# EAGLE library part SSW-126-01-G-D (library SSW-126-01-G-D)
52 Position, .100" Tiger Buy&trade; Socket Strip Source: Datasheet
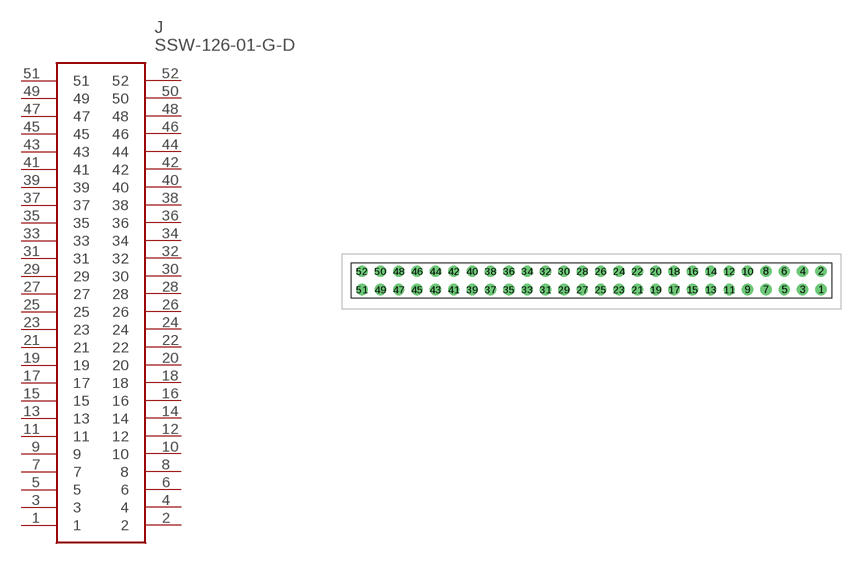
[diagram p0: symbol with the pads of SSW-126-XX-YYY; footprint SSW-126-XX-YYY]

Designator prefix J

## SSW-126-01-G-D (Description: 52 Position, .100&quot; Tiger Buy&trade; Socket Strip; Height: mm; Manufacturer_Name: SAMTEC; Manufacturer_Part_Number: SSW-126-01-G-D; Mouser_Part_Number: 200-SSW12601GD; Mouser_Price-Stock: https://www.mouser.co.uk/ProductDetail/Samtec/SSW-126-01-G-D?qs=rU5fayqh%252BE0Emlk%2F61GTGg%3D%3D)  [SSW-126-XX-YYY]
1  1
2  2
3  3
4  4
5  5
6  6
7  7
8  8
9  9
10  10
11  11
12  12
13  13
14  14
15  15
16  16
17  17
18  18
19  19
20  20
21  21
22  22
23  23
24  24
25  25
26  26
27  27
28  28
29  29
30  30
31  31
32  32
33  33
34  34
35  35
36  36
37  37
38  38
39  39
40  40
41  41
42  42
43  43
44  44
45  45
46  46
47  47
48  48
49  49
50  50
51  51
52  52

## Footprint SSW-126-XX-YYY (pad centres in mm)
SAMTEC_SSW-126-01-G-D
drill 1.04 pad 1.57: 1 0,0; 2 0,2.54; 3 -2.54,0; 4 -2.54,2.54; 5 -5.08,0; 6 -5.08,2.54; 7 -7.62,0; 8 -7.62,2.54; 9 -10.16,0; 10 -10.16,2.54; 11 -12.7,0; 12 -12.7,2.54; 13 -15.24,0; 14 -15.24,2.54; 15 -17.78,0; 16 -17.78,2.54; 17 -20.32,0; 18 -20.32,2.54; 19 -22.86,0; 20 -22.86,2.54; 21 -25.4,0; 22 -25.4,2.54; 23 -27.94,0; 24 -27.94,2.54; 25 -30.48,0; 26 -30.48,2.54; 27 -33.02,0; 28 -33.02,2.54; 29 -35.56,0; 30 -35.56,2.54; 31 -38.1,0; 32 -38.1,2.54; 33 -40.64,0; 34 -40.64,2.54; 35 -43.18,0; 36 -43.18,2.54; 37 -45.72,0; 38 -45.72,2.54; 39 -48.26,0; 40 -48.26,2.54; 41 -50.8,0; 42 -50.8,2.54; 43 -53.34,0; 44 -53.34,2.54; 45 -55.88,0; 46 -55.88,2.54; 47 -58.42,0; 48 -58.42,2.54; 49 -60.96,0; 50 -60.96,2.54; 51 -63.5,0; 52 -63.5,2.54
